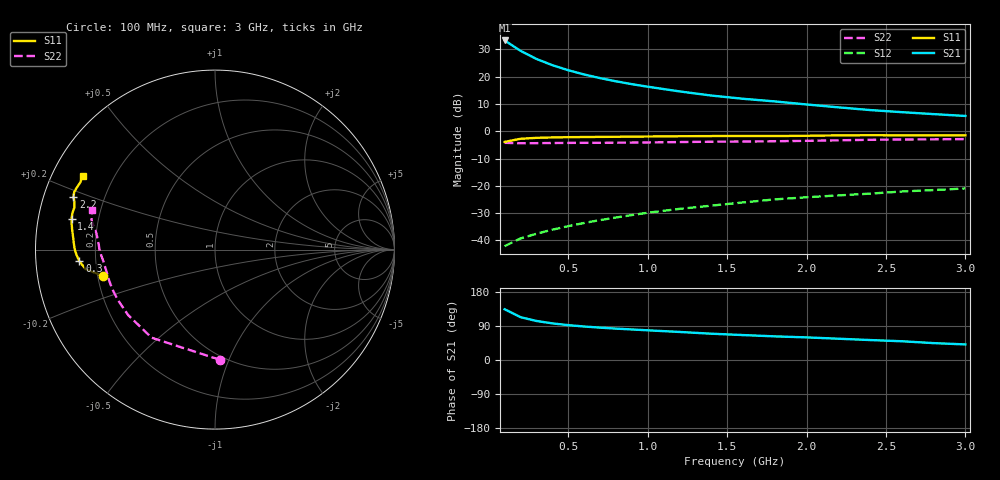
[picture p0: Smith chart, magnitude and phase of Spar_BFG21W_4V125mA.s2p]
! Filename: 4125bfg21.001
! Title: BFG21W
! Bias: Vce=4V; Ic=125mA
! Company: NXP Semiconductors NL
! User: Quality&Reliability T&D
! Measure time: 10 Nov 1999 / 11:45:57
#  MHz  S  MA  R 50
! Freq  S11  S21  S12  S22  :
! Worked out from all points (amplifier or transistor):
!   20 points, 100 MHz to 3 GHz, reference 50 ohm
!   highest |S21| = 33.3 dB at 100 MHz (marker M1)
!   |S21| within 3 dB of that: start of sweep to 179.1 MHz
!   unconditionally stable (mu >= 1): 624.7 MHz to end of sweep
!   at 400 MHz: K = 0.91, MSG = 30.2 dB, |S12| = -36.1 dB
!   at 1.2 GHz: K = 1.06, MAG = 20.0 dB, |S12| = -28.5 dB
!   at 3 GHz: K = 1.05, MAG = 11.9 dB, |S12| = -21.0 dB
!   S11 on the Smith chart (normalised r, x): 100 MHz: 0.22, -0.11; 300 MHz: 0.14, -0.04; 1.4 GHz: 0.10, +0.11; 2.2 GHz: 0.09, +0.18; 3 GHz: 0.09, +0.26
100  0.639 -166.6  46.27 133.9  0.007831 54.2  0.6141 -87.5
200  0.7291 -171.4  29.9 113.0  0.01086 52.7  0.6047 -125.7
300  0.7584 -175.1  21.23 103.0  0.01322 56.1  0.6059 -143.0
400  0.7717 -177.7  16.31 96.7  0.01568 59.6  0.6099 -152.6
500  0.7802 -179.8  13.19 92.0  0.01822 62.7  0.6127 -158.7
600  0.7851 178.4  11.01 88.4  0.02083 64.8  0.6143 -163.0
700  0.7891 176.8  9.455 85.4  0.02352 67.1  0.6153 -166.3
800  0.7928 175.2  8.253 82.8  0.02624 68.6  0.6173 -169.1
900  0.7974 173.8  7.319 80.6  0.02908 70.1  0.6206 -171.6
1000  0.8025 172.4  6.571 78.4  0.03212 70.8  0.6247 -173.7
1200  0.8114 169.8  5.39 74.0  0.0378 71.9  0.635 -177.2
1400  0.8174 167.8  4.525 69.4  0.04332 72.2  0.6438 179.9
1600  0.8201 165.7  3.949 65.8  0.04959 72.5  0.6487 177.3
1800  0.818 163.3  3.531 62.4  0.05642 72.6  0.6568 174.7
2000  0.8266 161.4  3.104 59.7  0.06176 73.0  0.6685 171.9
2200  0.8423 159.4  2.75 56.2  0.06676 72.8  0.6834 169.6
2400  0.8476 157.7  2.451 52.6  0.07196 71.9  0.6983 167.9
2600  0.8438 155.9  2.242 49.5  0.07873 70.8  0.708 166.4
2800  0.839 153.6  2.065 44.6  0.08368 69.1  0.7125 164.4
3000  0.8433 151.1  1.91 41.1  0.08958 68.1  0.7197 161.9
